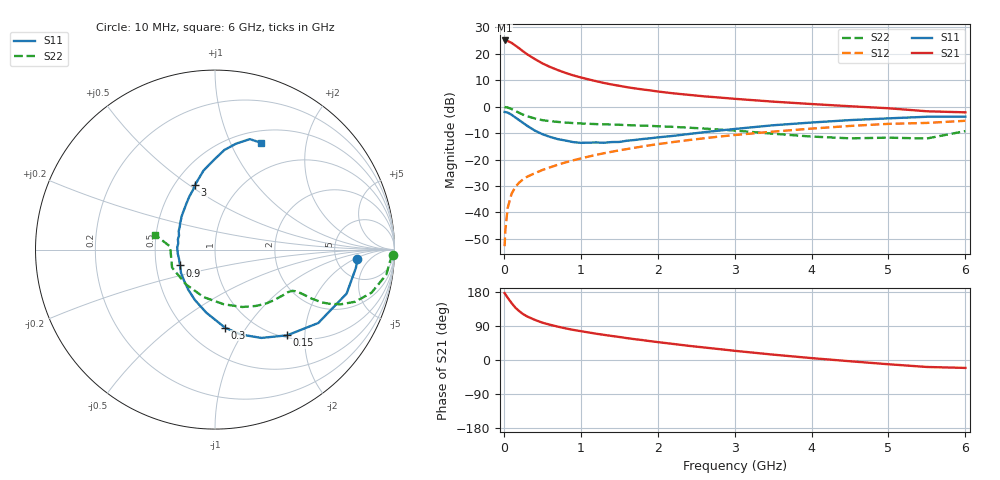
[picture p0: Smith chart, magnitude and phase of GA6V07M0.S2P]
! Infineon Technologies  Discrete & RF Semiconductors
! BF775
! Si NPN RF Bipolar Junction Transistor in SOT23
! VCE = 6 V  IC = 7 mA
! Common Emitter S-Parameters:  May  1996
# GHz  S  MA  R  50
!  f  S11  S21  S12  S22
! GHz  MAG  ANG  MAG  ANG  MAG  ANG  MAG  ANG
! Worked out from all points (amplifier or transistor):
!   36 points, 10 MHz to 6 GHz, reference 50 ohm
!   highest |S21| = 25.1 dB at 10 MHz (marker M1)
!   |S21| within 3 dB of that: start of sweep to 201.4 MHz
!   unconditionally stable (mu >= 1): 728.4 MHz to 3.032 GHz
!   at 250 MHz: K = 0.57, MSG = 24.2 dB, |S12| = -27.5 dB
!   at 1.4 GHz: K = 1.11, MAG = 10.8 dB, |S12| = -17.1 dB
!   at 6 GHz: K = 0.92, MSG = 1.6 dB, |S12| = -5.3 dB
!   S11 on the Smith chart (normalised r, x): 10 MHz: 8.16, -2.22; 150 MHz: 1.04, -1.63; 300 MHz: 0.75, -0.80; 900 MHz: 0.66, -0.12; 3 GHz: 0.63, +0.53; 6 GHz: 0.64, +1.31
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0.01  0.7952 -3.6  17.91 176.6  0.0023 87.5  0.9911 -1.7
0.02  0.7918 -7.3  17.62 173.3  0.0047 82.7  0.9792 -3.4
0.05  0.7731 -18.5  17.49 164.3  0.0122 81.6  0.9647 -8.3
0.1  0.7059 -35.4  16.16 150.5  0.0224 73.8  0.9044 -15.4
0.15  0.6244 -49.9  14.34 138.0  0.0305 67.3  0.8333 -20.4
0.2  0.5558 -62.3  12.72 128.9  0.0368 63.7  0.7644 -23.5
0.25  0.494 -73.2  11.16 121.2  0.0422 61.2  0.707 -25.3
0.3  0.4384 -82.7  9.878 115.2  0.0471 60.8  0.6642 -26.3
0.4  0.3549 -97.8  8.011 106.2  0.055 60.1  0.601 -26.9
0.5  0.3028 -111.6  6.62 98.6  0.0634 60.8  0.5572 -26.9
0.6  0.2686 -123.7  5.655 93.0  0.0712 61.1  0.5327 -27.0
0.7  0.2437 -135.2  4.94 88.1  0.0797 61.6  0.5157 -27.2
0.9  0.2141 -155.7  3.924 79.5  0.0966 62.1  0.4903 -27.9
1.1  0.2087 -173.8  3.288 72.7  0.1137 62.5  0.4752 -29.7
1.3  0.2077 170.4  2.815 66.4  0.1317 61.9  0.4633 -31.7
1.6  0.2272 152.9  2.341 57.7  0.158 60.5  0.4486 -35.8
2.2  0.2804 128.1  1.792 42.4  0.2143 56.4  0.4158 -45.9
3  0.379 106.9  1.41 24.3  0.291 48.7  0.354 -64.6
3.5  0.4455 98.2  1.247 14.2  0.3378 43.0  0.3082 -81.0
4.5  0.5578 84.6  1.02 -3.3  0.4324 30.5  0.2523 -129.9
5.5  0.6454 72.5  0.819 -18.4  0.4933 15.4  0.2504 176.1
6  0.6475 66.9  0.782 -20.9  0.5414 11.3  0.3458 166.0
